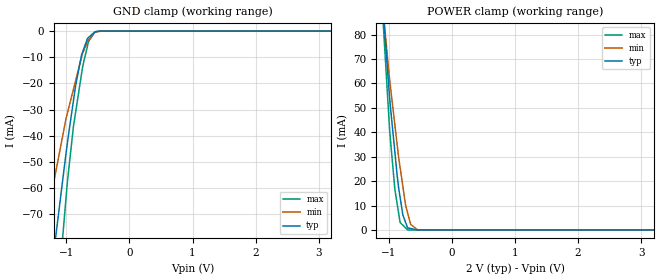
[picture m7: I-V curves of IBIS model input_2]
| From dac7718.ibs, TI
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|   input_2 Model
[Model]   input_2
Model_type   Input
Vinl = 0.3
Vinh = 1.5
|   typ   min   max
|   (nom PVT)   (Fast PVT)   (slow PVT)
|C_comp from frequency method(F=50MHz)
|Average
C_comp   9.478e-12   7.793e-12   1.106e-11
|C_comp from LC tank method(L=1nH)
|Resonant Frequency(Hz)   1.71e9   1.86e9   1.59e9
|C_comp   8.671e-12   7.329e-12   1.003e-11
| Where nom  PVT is Nominal Process,  2V,  33C
|   Fast PVT is Strong Process,   2.2V,  -40C
|   Slow PVT is Weak Process,   1.8V,  113C
[Voltage Range]   2   1.8   2.2
|Ambient Temperature   25   85   -40
|Junction Temperature
[Temperature Range]   33   113   -40
[Power Clamp Reference]   2   1.8   2.2
[GND Clamp Reference]   0   0   0
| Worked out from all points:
|   GND clamp passes 1 mA (typ) near -0.58 V on its own axis
|   POWER clamp passes 1 mA (typ) near -0.71 V on its own axis
[GND Clamp]
|   Voltage   I(typ)   I(min)   I(max)
-2V       -263.5mA   -170mA     -377.7mA
-1.37V    -120.8mA   -78.93mA   -174.1mA
-1.305V   -107mA     -70.77mA   -153.1mA
-1.166V   -77.82mA   -53.43mA   -110mA
-1.115V   -67.95mA   -47.1mA    -94.69mA
-1.008V   -47.01mA   -33.66mA   -64.24mA
-983.4mV  -42.49mA   -31.28mA   -57.37mA
-888.8mV  -26.6mA    -22.25mA   -36.46mA
-762mV    -9.323mA   -10.15mA   -16.61mA
-649mV    -2.441mA   -3.363mA   -3.943mA
-550mV    -287.9uA   -547.7uA   -411.5uA
4V        0A         0A         0A
[POWER Clamp]
|   Voltage   I(typ)   I(min)   I(max)
-2V       432.1mA    366.4mA    517.3mA
-1.133V   103.9mA    101.2mA    102.8mA
-993.6mV  55.71mA    62.67mA    42.93mA
-906.4mV  32.05mA    43.15mA    16.74mA
-868mV    21.94mA    34.59mA    10.44mA
-822.8mV  13.36mA    25.58mA    3.031mA
-778mV    6.055mA    17.64mA    1.896mA
-736.2mV  3.12mA     10.24mA    837.5uA
-704mV    860uA      7.032mA    21.8uA
-655.2mV  588.5uA    2.293mA    14.91uA
-518.4mV  1.087uA    51.2uA     29.1nA
4V        0A         0A         0A
